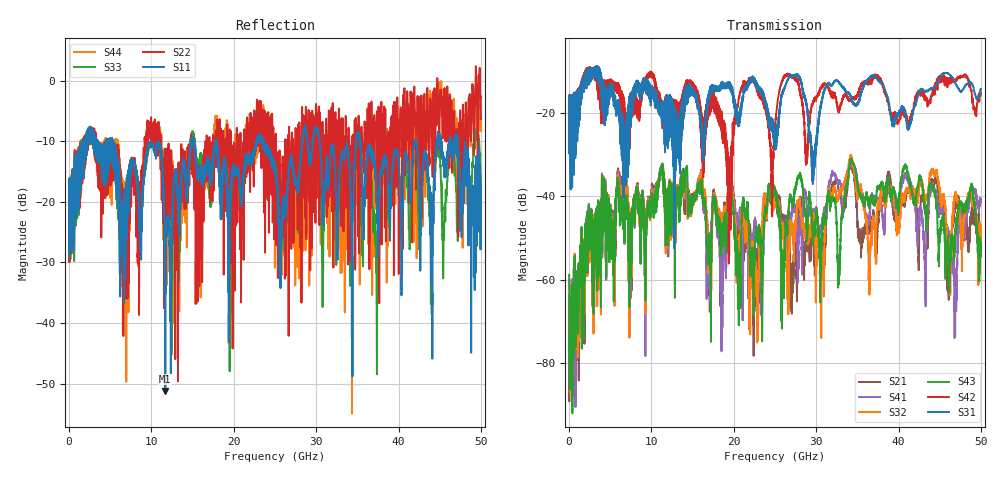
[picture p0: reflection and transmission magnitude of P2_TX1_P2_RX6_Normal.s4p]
!Keysight Technologies,N5225B,MY57041031,A.13.20.10
!Date: Friday, May 31, 2019 11:35:47
!Correction: S11(Full 4 Port(1,2,3,4))
!S12(Full 4 Port(1,2,3,4))
!S13(Full 4 Port(1,2,3,4))
!S14(Full 4 Port(1,2,3,4))
!S21(Full 4 Port(1,2,3,4))
!S22(Full 4 Port(1,2,3,4))
!S23(Full 4 Port(1,2,3,4))
!S24(Full 4 Port(1,2,3,4))
!S31(Full 4 Port(1,2,3,4))
!S32(Full 4 Port(1,2,3,4))
!S33(Full 4 Port(1,2,3,4))
!S34(Full 4 Port(1,2,3,4))
!S41(Full 4 Port(1,2,3,4))
!S42(Full 4 Port(1,2,3,4))
!S43(Full 4 Port(1,2,3,4))
!S44(Full 4 Port(1,2,3,4))
!S4P File: Measurements: <S11,S12,S13,S14>,
!<S21,S22,S23,S24>,
!<S31,S32,S33,S34>,
!<S41,S42,S43,S44>:
# Hz S  dB  R 50.0
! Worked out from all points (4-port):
!   5000 points, 10 MHz to 50 GHz, reference 50 ohm
!   strongest paths, dB at 10 MHz, 12.51 GHz, 25.01 GHz, 37.51 GHz, 50 GHz:
!     S31: -19.5, -17.3, -28.8, -12.1, -14.2
!     S42: -19.4, -16.6, -23.5, -10.9, -15.1
!     S43: -58.9, -37.5, -38.2, -37.7, -51.2
!     S32: -64.7, -37.0, -41.4, -41.7, -47.0
!     S41: -63.7, -38.7, -38.9, -40.7, -40.6
!     S21: -65.0, -37.9, -40.9, -46.0, -51.2
!   lowest |S11| = -51.2 dB at 11.69 GHz (marker M1), VSWR 1.01, Z = 49.8 - j0.171 ohm
!   |S11| at or under -10 dB: 5.36 GHz to 10.81 GHz (5.449 GHz wide, 67.4 % of centre); 17.89 GHz to 22.7 GHz (4.805 GHz wide, 23.7 % of centre); 35.31 GHz to 41.96 GHz (6.644 GHz wide, 17.2 % of centre)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
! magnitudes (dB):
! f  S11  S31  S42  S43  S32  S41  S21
! 10 MHz  -19.5  -19.5  -19.4  -58.9  -64.7  -63.7  -65.0
! 11.69 GHz  -51.2  -23.0  -18.9  -46.8  -47.4  -47.6  -47.9
! 22.76 GHz  -10.2  -13.8  -13.2  -47.4  -61.1  -47.8  -53.9
! 24.36 GHz  -12.4  -23.5  -24.9  -38.8  -38.9  -38.4  -37.4
! 40.87 GHz  -12.4  -20.5  -20.3  -32.8  -39.3  -35.3  -40.9
! 46.89 GHz  -10.2  -12.7  -12.0  -47.8  -39.9  -58.8  -42.3
! 50 GHz  -17.3  -14.2  -15.1  -51.2  -47.0  -40.6  -51.2
